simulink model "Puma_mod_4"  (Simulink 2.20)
settings: Solver=VariableStepDiscrete  StartTime=0.0  StopTime=10.0  RelTol=1e-3  AbsTol=1e-6

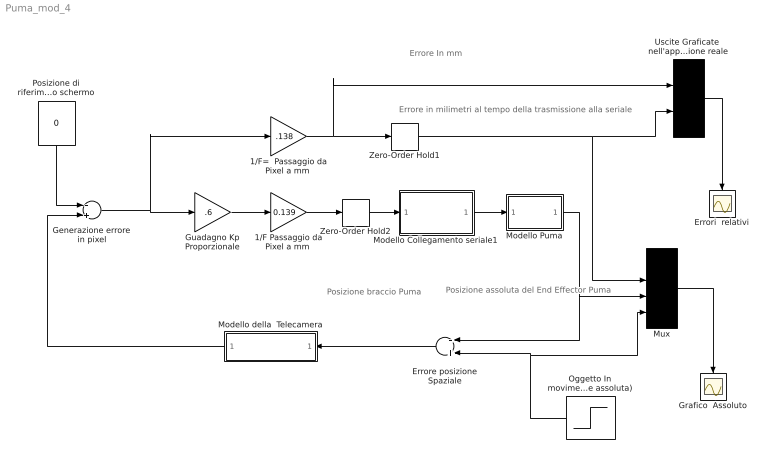
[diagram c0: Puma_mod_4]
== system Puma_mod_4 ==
  note: Posizione braccio Puma
  note: Posizione assoluta del End Effector Puma
  note: Errore In mm
  note: Errore in milimetri al tempo della trasmissione alla seriale
  "1/F Passaggio da Pixel a mm " : Gain  Gain=0.139
  "1/F=  Passaggio da Pixel a mm " : Gain  Gain=.138
  Errore posizione Spaziale : Sum  Orientation=left  Inputs=-+
  Errori  relativi : Scope
  Generazione errore in pixel : Sum  Inputs=-+
  Grafico  Assoluto : Scope
  Guadagno Kp Proporzionale : Gain  Gain=.6
  Modello Collegamento seriale1 : Subsystem  Description=Modello seriale
  Modello Puma : Subsystem  Description=Modello Puma
  Modello della  Telecamera : Subsystem  Orientation=left
  Mux : Mux  Inputs=4
  Oggetto In movimento ( posizione assoluta) : Step  Orientation=left  Time=.010  Before=0  After=48.5
  Posizione di riferimento  nello schermo : Constant  Orientation=down  Value=0
  Uscite Graficate  nell'applicazione reale : Mux  Inputs=2
  Zero-Order Hold1 : ZeroOrderHold  SampleTime=.250
  Zero-Order Hold2 : ZeroOrderHold  SampleTime=.250
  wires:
  Mux/1 -> Grafico  Assoluto/1
  Posizione di riferimento  nello schermo/1 -> Generazione errore in pixel/1
  Guadagno Kp Proporzionale/1 -> "1/F Passaggio da Pixel a mm "/1
  Oggetto In movimento ( posizione assoluta)/1 -> Errore posizione Spaziale/2, Mux/4
  Generazione errore in pixel/1 -> Guadagno Kp Proporzionale/1, "1/F=  Passaggio da Pixel a mm "/1
  Uscite Graficate  nell'applicazione reale/1 -> Errori  relativi/1
  Zero-Order Hold1/1 -> Mux/2, Uscite Graficate  nell'applicazione reale/2
  "1/F Passaggio da Pixel a mm "/1 -> Zero-Order Hold2/1
  Zero-Order Hold2/1 -> Modello Collegamento seriale1/1(In1)
  Modello Collegamento seriale1/1(Out1) -> Modello Puma/1(In1)
  "1/F=  Passaggio da Pixel a mm "/1 -> Zero-Order Hold1/1, Uscite Graficate  nell'applicazione reale/1
  Errore posizione Spaziale/1 -> Modello della  Telecamera/1(In1)
  Modello della  Telecamera/1(Out1) -> Generazione errore in pixel/2
  Modello Puma/1(Out1) -> Errore posizione Spaziale/1, Mux/3

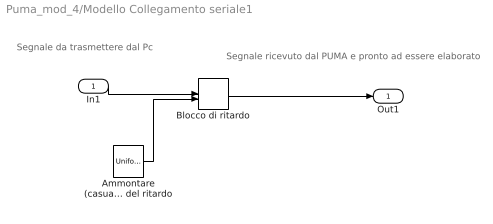
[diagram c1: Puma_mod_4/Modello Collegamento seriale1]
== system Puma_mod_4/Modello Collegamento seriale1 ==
  note: Segnale da trasmettere dal Pc
  note: Segnale ricevuto dal PUMA e pronto ad essere elaborato
  In1 : Inport  Port=1  PortWidth=-1  SampleTime=-1
  Ammontare (casuale)  in ms del ritardo : UniformRandomNumber  Minimum=.260  Maximum=.290  Seed=0  SampleTime=.280
  Blocco di ritardo : VariableTransportDelay  MaximumDelay=1  InitialInput=0  MaximumPoints=1024
  Out1 : Outport  Port=1
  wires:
  Ammontare (casuale)  in ms del ritardo/1 -> Blocco di ritardo/2
  In1/1 -> Blocco di ritardo/1
  Blocco di ritardo/1 -> Out1/1

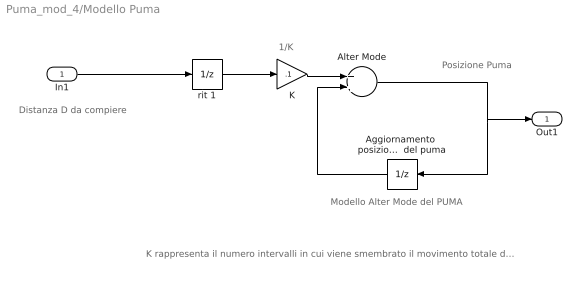
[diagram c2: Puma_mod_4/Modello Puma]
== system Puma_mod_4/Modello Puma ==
  note: Posizione Puma
  note: Modello Alter Mode del PUMA
  note: 1/K
  note: K rappresenta il numero intervalli in cui viene smembrato il movimento totale da compiere, dopo K time-slice (del PUMA) si ottiene che si e' compiuto proprio la distanza D trasmessa.
  note: Distanza D da compiere
  In1 : Inport  Port=1  PortWidth=-1  SampleTime=-1
  Aggiornamento  posizione   Il sample-time di questo blocco rappresenta la TIME-SLICE  del puma : UnitDelay  Orientation=left  X0=0  SampleTime=.034
  Alter Mode : Sum  Inputs=++
  K : Gain  Gain=.1
  rit 1 : UnitDelay  X0=0  SampleTime=.034
  Out1 : Outport  Port=1
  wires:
  Alter Mode/1 -> Aggiornamento  posizione   Il sample-time di questo blocco rappresenta la TIME-SLICE  del puma/1, Out1/1
  K/1 -> Alter Mode/1
  Aggiornamento  posizione   Il sample-time di questo blocco rappresenta la TIME-SLICE  del puma/1 -> Alter Mode/2
  rit 1/1 -> K/1
  In1/1 -> rit 1/1

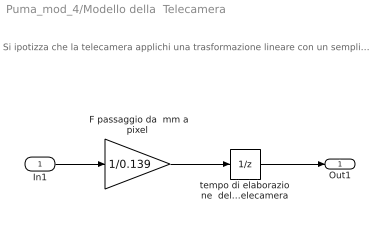
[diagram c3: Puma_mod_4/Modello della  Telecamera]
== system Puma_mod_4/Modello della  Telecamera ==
  note: Si ipotizza che la telecamera applichi una trasformazione lineare con un semplice fattore di scala F. ( ricavato automaticamente dalla procedura di calibrazione)
  In1 : Inport  Port=1  PortWidth=-1  SampleTime=-1
  " F passaggio da  mm a pixel" : Gain  Gain=1/0.139
  tempo di elaborazione  della telecamera : UnitDelay  X0=0  SampleTime=.033
  Out1 : Outport  Port=1
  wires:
  In1/1 -> " F passaggio da  mm a pixel"/1
  " F passaggio da  mm a pixel"/1 -> tempo di elaborazione  della telecamera/1
  tempo di elaborazione  della telecamera/1 -> Out1/1
